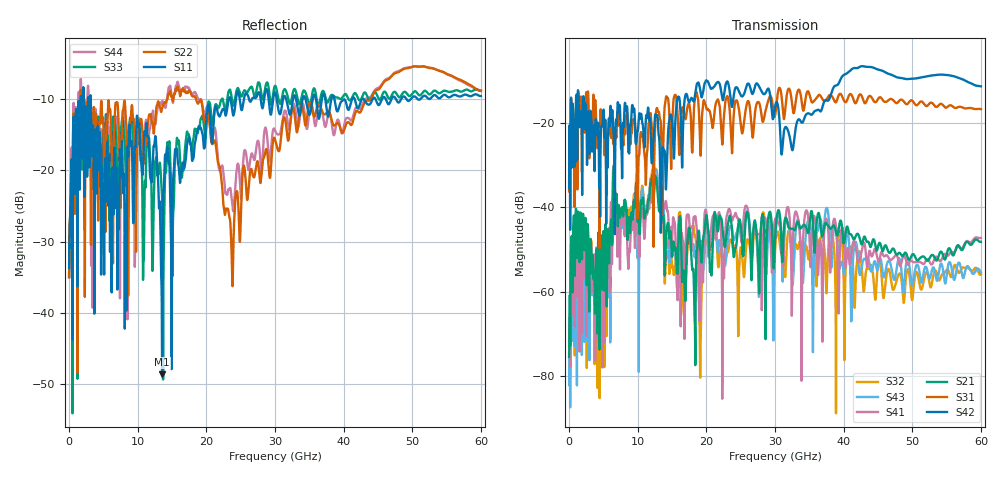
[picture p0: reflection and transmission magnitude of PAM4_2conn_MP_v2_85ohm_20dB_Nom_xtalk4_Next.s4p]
! Info: Touchstone file created by Circ.  Input file=FAB50GbE_2conn_Midplane_Examax_Topo2_v2_85ohm_20dB_Nom.circ
# Hz S RI R 50
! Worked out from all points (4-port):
!   6000 points, 10 MHz to 60 GHz, reference 50 ohm
!   strongest paths, dB at 10 MHz, 15.01 GHz, 30.01 GHz, 45.01 GHz, 60 GHz:
!     S42: -35.6, -19.6, -16.3, -7.5, -11.4
!     S31: -36.3, -21.1, -18.4, -14.5, -16.8
!     S21: -75.4, -51.6, -47.5, -49.4, -48.2
!     S41: -68.0, -48.0, -42.9, -52.6, -47.3
!     S43: -71.0, -51.2, -47.6, -54.5, -55.4
!     S32: -74.7, -54.0, -50.5, -53.5, -55.9
!   lowest |S11| = -48.6 dB at 13.55 GHz (marker M1), VSWR 1.01, Z = 50.2 + j0.288 ohm
!   |S11| at or under -10 dB: start of sweep to 1.704 GHz; 3.16 GHz to 23.24 GHz (20.08 GHz wide, 152 % of centre); 38.66 GHz to 41.24 GHz (2.581 GHz wide, 6.46 % of centre)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
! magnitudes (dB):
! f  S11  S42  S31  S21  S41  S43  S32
! 10 MHz  -33.7  -35.6  -36.3  -75.4  -68.0  -71.0  -74.7
! 1.19 GHz  -29.4  -27.6  -29.3  -52.0  -55.5  -58.6  -56.7
! 13.55 GHz  -48.6  -28.4  -31.0  -43.0  -39.4  -40.2  -41.5
! 18.15 GHz  -18.1  -15.0  -18.3  -56.0  -42.4  -49.1  -44.8
! 19.08 GHz  -14.0  -12.1  -23.8  -49.8  -57.2  -58.2  -76.6
! 23.76 GHz  -11.4  -16.3  -27.1  -45.7  -43.2  -45.4  -48.3
! 60 GHz  -9.6  -11.4  -16.8  -48.2  -47.3  -55.4  -55.9
